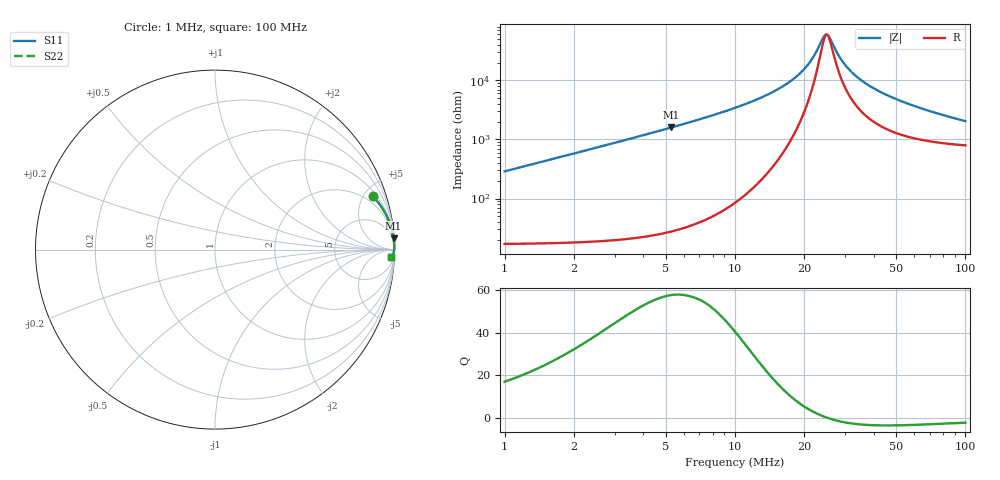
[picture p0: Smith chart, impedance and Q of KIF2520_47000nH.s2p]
!version-2
!date-12.2020
!Series
# MHz S RI R 50
!Freq ReS11 ImS11 ReS21 ImS21 ReS12 ImS12 ReS22 ImS22
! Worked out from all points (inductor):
!   991 points, 1 MHz to 100 MHz, reference 50 ohm
!   read as one part in series: L = 45.8 uH near 1.4 MHz
!   highest Q = 57.4 at 5.3 MHz (marker M1), where L = 47.9 uH
!   self-resonance near 25 MHz
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1  0.8789 0.298  0.1211 -0.298  0.1211 -0.298  0.8789 0.298
2  0.9662 0.1659  0.0338 -0.1659  0.0338 -0.1659  0.9662 0.1659
2.8  0.9824 0.1201  0.0176 -0.1201  0.0176 -0.1201  0.9824 0.1201
3.9  0.9909 0.086  0.00913 -0.086  0.00913 -0.086  0.9909 0.086
5.3  0.995 0.0623  0.00498 -0.0623  0.00498 -0.0623  0.995 0.0623
8.4  0.9979 0.0366  0.00209 -0.0366  0.00209 -0.0366  0.9979 0.0366
17.5  0.9989 0.0101  0.00113 -0.0101  0.00113 -0.0101  0.9989 0.0101
20.8  0.9987 0.00517  0.0013 -0.00517  0.0013 -0.00517  0.9987 0.00517
22.2  0.9986 0.00335  0.00141 -0.00335  0.00141 -0.00335  0.9986 0.00335
24.1  0.9984 0.00108  0.00158 -0.00108  0.00158 -0.00108  0.9984 0.00108
24.9  0.9983 0.000189  0.00166 -0.000189  0.00166 -0.000189  0.9983 0.000189
25.6  0.9983 -0.00057  0.00173 0.00057  0.00173 0.00057  0.9983 -0.00057
27.8  0.998 -0.00283  0.00198 0.00283  0.00198 0.00283  0.998 -0.00283
29.5  0.9978 -0.00445  0.00219 0.00445  0.00219 0.00445  0.9978 -0.00445
31.5  0.9975 -0.00626  0.00247 0.00626  0.00247 0.00626  0.9975 -0.00626
34  0.9972 -0.00839  0.00283 0.00839  0.00283 0.00839  0.9972 -0.00839
37.1  0.9967 -0.0109  0.00333 0.0109  0.00333 0.0109  0.9967 -0.0109
40.8  0.996 -0.0136  0.00399 0.0136  0.00399 0.0136  0.996 -0.0136
50.5  0.994 -0.02  0.00598 0.02  0.00598 0.02  0.994 -0.02
67  0.9898 -0.0293  0.0102 0.0293  0.0102 0.0293  0.9898 -0.0293
83.5  0.9849 -0.037  0.0151 0.037  0.0151 0.037  0.9849 -0.037
100  0.9794 -0.0434  0.0206 0.0434  0.0206 0.0434  0.9794 -0.0434
